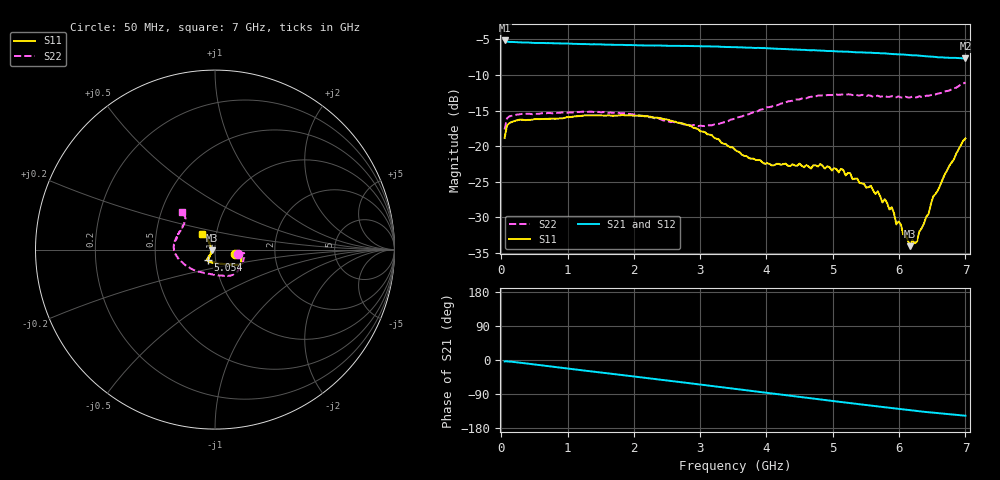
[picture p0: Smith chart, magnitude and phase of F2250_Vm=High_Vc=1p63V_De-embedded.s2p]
! Integrated Device Technology
! Corporate Headquarters
! 6024 Silver Creek Valley Road
! San Jose, CA 95138  USA
! Phone:  1-408-284-8200
! Toll Free:  1-800-223-1366
! Webpage:  http://www.idt.com/
! Timing and RF Division
! 515 Groton Road, Suite 102
! Westford, MA 01886-6024
! Device:  F2250
! Description: Voltage Variable RF Attenuator
! Frequency:  50.0 -  6000.00 MHz
! Package:  3x3 mm Thin QFN Plastic Package: 16 pin
! Ports:  2 RF, 3 DC
!  Pin  1  = GND
!  Pin  2  = NC
!  Pin  3  = RF1  = Port 1
!  Pin  4  = NC
!  Pin  5  = GND
!  Pin  6  = GND
!  Pin  7  = GND
!  Pin  8  = GND
!  Pin  9  = NC
!  Pin 10  = RF2  = Port 2
!  Pin 11  = NC
!  Pin 12  = GND
!  Pin 13  = GND
!  Pin 14  = VCNTRL
!  Pin 15  = VDD
!  Pin 16  = VMODE
! Vcntrl:  1.630 Volts
! Vmode:  +3.300 Volts
! Vdd:  +3.30  Volts
! Current:  1.328 mA
! Data:  The device was measured on a the F2250 evaluation board which has
!  individual transmission lines to the RF pins.  Data was collected
!  using a calibrated network analyzer.  The evaluation board was
!  de-embedded using a TRL calibration technique.
!  The reference plane is the edge of the package pin.
! Misc:  SN 10
!  Action Tracker AT0258
! Date Measured:  2014-11-26
! Date:  2015-10-15  MJV
! Note:
!  Integrated Device Technology supplies this data as a sample of measured
!  data at the package pin for this product.  Your particular data for this
!  product may vary.
!  Data was taken at 25 degrees C.
!  Integrated Device Technology reserves the right to change this data at anytime.
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# GHz S dB R 50
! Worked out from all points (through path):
!   201 points, 50 MHz to 7 GHz, reference 50 ohm
!   highest |S21| = -5.15 dB at 50 MHz (marker M1); lowest = -7.7 dB at 7 GHz (marker M2)
!   group delay of S21, straight-line fit = 59 ps
!   lowest |S11| = -34.0 dB at 6.166 GHz (marker M3), VSWR 1.04, Z = 48.1 - j0.402 ohm
!   |S11| at or under -10 dB: start of sweep to end of sweep
!   |S22| runs from -17.7 to -11.1 dB; largest |S21 - S12| = 0.0023
!   S11 on the Smith chart (normalised r, x): 50 MHz: 1.25, -0.06; 5.054 GHz: 0.92, -0.11; 7 GHz: 0.85, +0.15
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0.05  -18.85 -11.9  -5.15 -3.7  -5.15 -3.7  -17.65 -10.9
0.08475  -17.13 -6.8  -5.30 -3.6  -5.32 -3.6  -16.11 -7.1
0.2585  -16.30 -7.9  -5.41 -6.6  -5.42 -6.6  -15.55 -11.5
1.2315  -15.71 -26.7  -5.66 -27.4  -5.64 -27.4  -15.15 -43.1
2.37825  -16.04 -33.4  -5.85 -51.3  -5.87 -51.4  -16.13 -70.8
2.969  -17.63 -38.9  -5.96 -64.1  -5.95 -64.1  -17.19 -96.9
3.525  -20.50 -58.3  -6.09 -76.4  -6.07 -76.4  -16.13 -129.5
4.081  -22.71 -92.3  -6.28 -88.6  -6.31 -88.6  -14.42 -155.2
4.7065  -22.68 -121.1  -6.51 -102.0  -6.52 -102.0  -13.07 -173.8
5.054  -23.21 -124.5  -6.69 -109.4  -6.68 -109.4  -12.73 177.8
5.57525  -25.57 -129.5  -6.87 -120.2  -6.87 -120.3  -12.92 165.6
5.85325  -28.91 -134.3  -7.02 -126.0  -7.02 -126.1  -13.07 157.0
5.888  -28.58 -136.3  -7.05 -126.8  -7.03 -126.9  -12.96 157.0
5.9575  -30.98 -138.0  -7.08 -128.1  -7.06 -128.3  -13.13 154.2
6.027  -31.00 -146.6  -7.11 -129.6  -7.09 -129.7  -13.16 152.8
6.166  -34.05 -167.9  -7.21 -132.4  -7.19 -132.5  -13.15 147.7
6.20075  -33.20 179.9  -7.23 -133.2  -7.22 -133.3  -13.02 147.0
6.27025  -33.39 165.3  -7.24 -134.6  -7.27 -134.6  -13.13 144.3
6.305  -31.98 153.4  -7.29 -135.3  -7.28 -135.4  -12.98 143.3
6.444  -29.54 137.1  -7.39 -137.9  -7.38 -138.0  -12.92 139.2
6.5135  -27.08 131.5  -7.43 -139.1  -7.43 -139.3  -12.77 136.9
7  -18.92 129.7  -7.66 -147.1  -7.67 -147.2  -11.06 130.8
